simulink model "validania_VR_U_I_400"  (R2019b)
settings: Solver=VariableStepAuto  StartTime=0.0  StopTime=10.0  RelTol=1e-3
libraries: powerlib x8

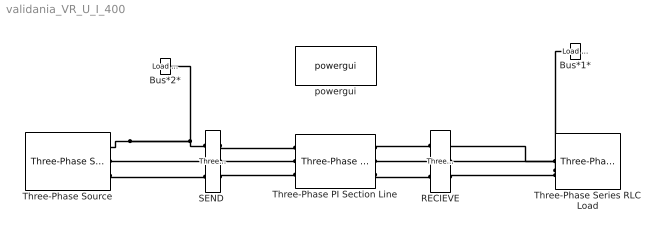
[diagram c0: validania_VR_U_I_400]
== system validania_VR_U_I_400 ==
  Bus*1* : powerlib/Measurements/Load Flow Bus  LConnTagsString=a  Phases=single  Connectors=on one side  ID=Bus*1*  Vbase=400000  Vref=1  Vangle=0  VLF=1.027  VLFb=1  VLFc=1  angleLF=-4.555  angleLFb=0  angleLFc=0
  Bus*2* : powerlib/Measurements/Load Flow Bus  LConnTagsString=a  Phases=single  Connectors=on one side  ID=Bus*2*  Vbase=413000  Vref=1  Vangle=0  VLF=1  VLFb=1  VLFc=1  angleLF=0  angleLFb=0  angleLFc=0
  RECIEVE : powerlib/Measurements/Three-Phase V-I Measurement  VoltageMeasurement=phase-to-phase  SetLabelV=on  LabelV=Vabc_R  Vpu=off  VpuLL=off  CurrentMeasurement=yes  SetLabelI=on  LabelI=Iabc_R  Ipu=off  Pbase=100e6  Vbase=500e3  OutputType=Complex  PhasorSimulation=off  PSBequivalent=0
  "SEND " : powerlib/Measurements/Three-Phase V-I Measurement  VoltageMeasurement=phase-to-phase  SetLabelV=on  LabelV=Vabc  Vpu=off  VpuLL=off  CurrentMeasurement=yes  SetLabelI=on  LabelI=Iabc  Ipu=off  Pbase=100e6  Vbase=500e3  OutputType=Complex  PhasorSimulation=off  PSBequivalent=0
  Three-Phase PI Section Line : powerlib/Elements/Three-Phase PI Section Line  LConnTagsString=a|b|c  RConnTagsString=A|B|C  Frequency=50  Resistances=[ 0.0259622 0.157407]  Inductances="[ 0.853601e-3  2.02405e-3]"  Capacitances=[13.4565e-9 7.54056e-9]  Length=100
  Three-Phase Series RLC Load : powerlib/Elements/Three-Phase Series RLC Load  LConnTagsString=A|B|C  Configuration=Y (grounded)  NominalVoltage=(400000)  Vabc=[1e3 1e3 1e3]  Vabcp=[1e3 1e3 1e3]  NominalFrequency=50  UnbalancedPower=off  ActivePower=500e6  InductivePower=0  CapacitivePower=0  Pabc=[10e3 9e3 11e3]  QLabc=[100 90 110]  QCabc=[100 90 110]  Pabcp=[10e3 9e3 11e3]  QLabcp=[100 90 110]  QCabcp=[100 90 110]  Measurements=Branch voltages and currents  LoadType=constant Z
  Three-Phase Source : powerlib/Electrical Sources/Three-Phase Source  InternalConnection=Yg  VoltagePhases=off  Voltage=(413000)*1  PhaseAngle=8.8158e-07  Voltage_phases=[25e3 25e3 25e3]/sqrt(3)  PhaseAngles_phases=[0 -120 +120]  Frequency=50  NonIdealSource=on  SpecifyImpedance=off  Resistance=0.000000001  Inductance=16.58e-9  ShortCircuitLevel=100e6  BaseVoltage=413e3  XRratio=7  BusType=swing  Pref=10e3  Qref=0  Prefabc=[10e3, 10e3, 10e3]  Qrefabc=[0, 0, 0]  Qmin=-inf  Qmax=inf
  powergui : powerlib/powergui  Priority=1  SimulationMode=Continuous  SampleTime=50e-6  frequency=60  Iterations=50  frequencyindice=50  Pbase=100e6  ErrMax=0.0001  UnitsV=kV  UnitsW=MW  buscounter=2  FunctionMessages=off  echomessages=off  EnableUseOfTLC=off  CurrentSourceSwitches=off  DisableSnubberDevices=off  DisableRonSwitches=off  DisableVfSwitches=off  DisplayEquations=off  AutomaticDiscreteSolvers=off  SolverType=Tustin/Backward Euler (TBE)  Interpol=off  ExternalGateDelay=off  methode=off  Ts=100  x0status=blocks  SPID=on  SwTol=0  HookPort=off  NonlinearTolerance=1e-4  nMaxIteration=100  ContinueOnMaxIteration=off  RestoreLinks=warning  ResistiveCurrentMeasurement=off  Frange=[0:2:500]  Ylog=off  Xlog=on  ShowGrid=off  save=off  variable=ZData  structure=0  ZoomFFT=off  StartTime=0.0  cycles=1  DisplayStyle=1  fundamental=60  FreqAxis=off  MaxFrequency=1000  frequencyindicesteady=1  RmsSteady=2  display=off
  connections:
  "SEND "/LConn1 -- Bus*2*/LConn1 -- Three-Phase Source/RConn1
  Three-Phase Source/RConn2 -- "SEND "/LConn2
  Three-Phase Source/RConn3 -- "SEND "/LConn3
  "SEND "/RConn1 -- Three-Phase PI Section Line/LConn1
  "SEND "/RConn2 -- Three-Phase PI Section Line/LConn2
  "SEND "/RConn3 -- Three-Phase PI Section Line/LConn3
  Three-Phase PI Section Line/RConn1 -- RECIEVE/LConn1
  Three-Phase PI Section Line/RConn2 -- RECIEVE/LConn2
  Three-Phase PI Section Line/RConn3 -- RECIEVE/LConn3
  Three-Phase Series RLC Load/LConn1 -- Bus*1*/LConn1 -- RECIEVE/RConn1
  Three-Phase Series RLC Load/LConn2 -- RECIEVE/RConn2
  RECIEVE/RConn3 -- Three-Phase Series RLC Load/LConn3
